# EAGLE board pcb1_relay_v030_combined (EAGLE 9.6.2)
2024-07-10 PCB made by JLCPCB.
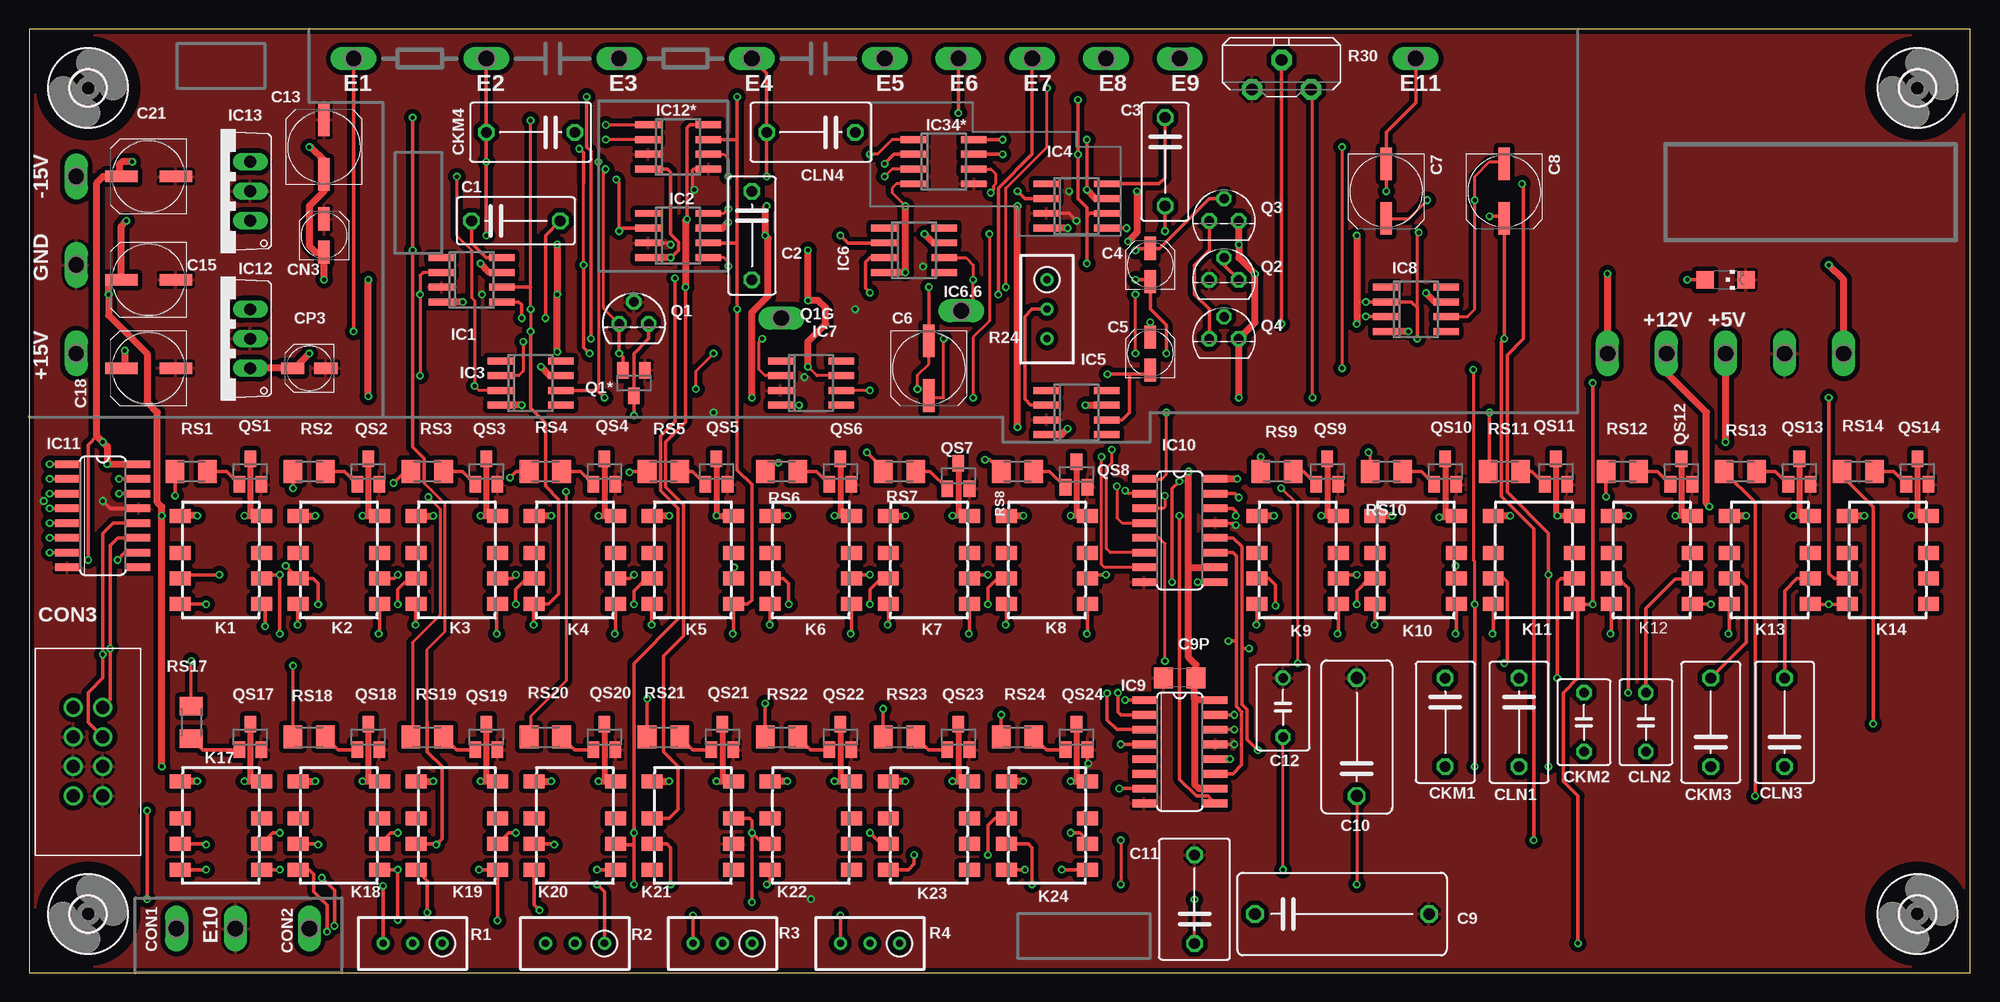
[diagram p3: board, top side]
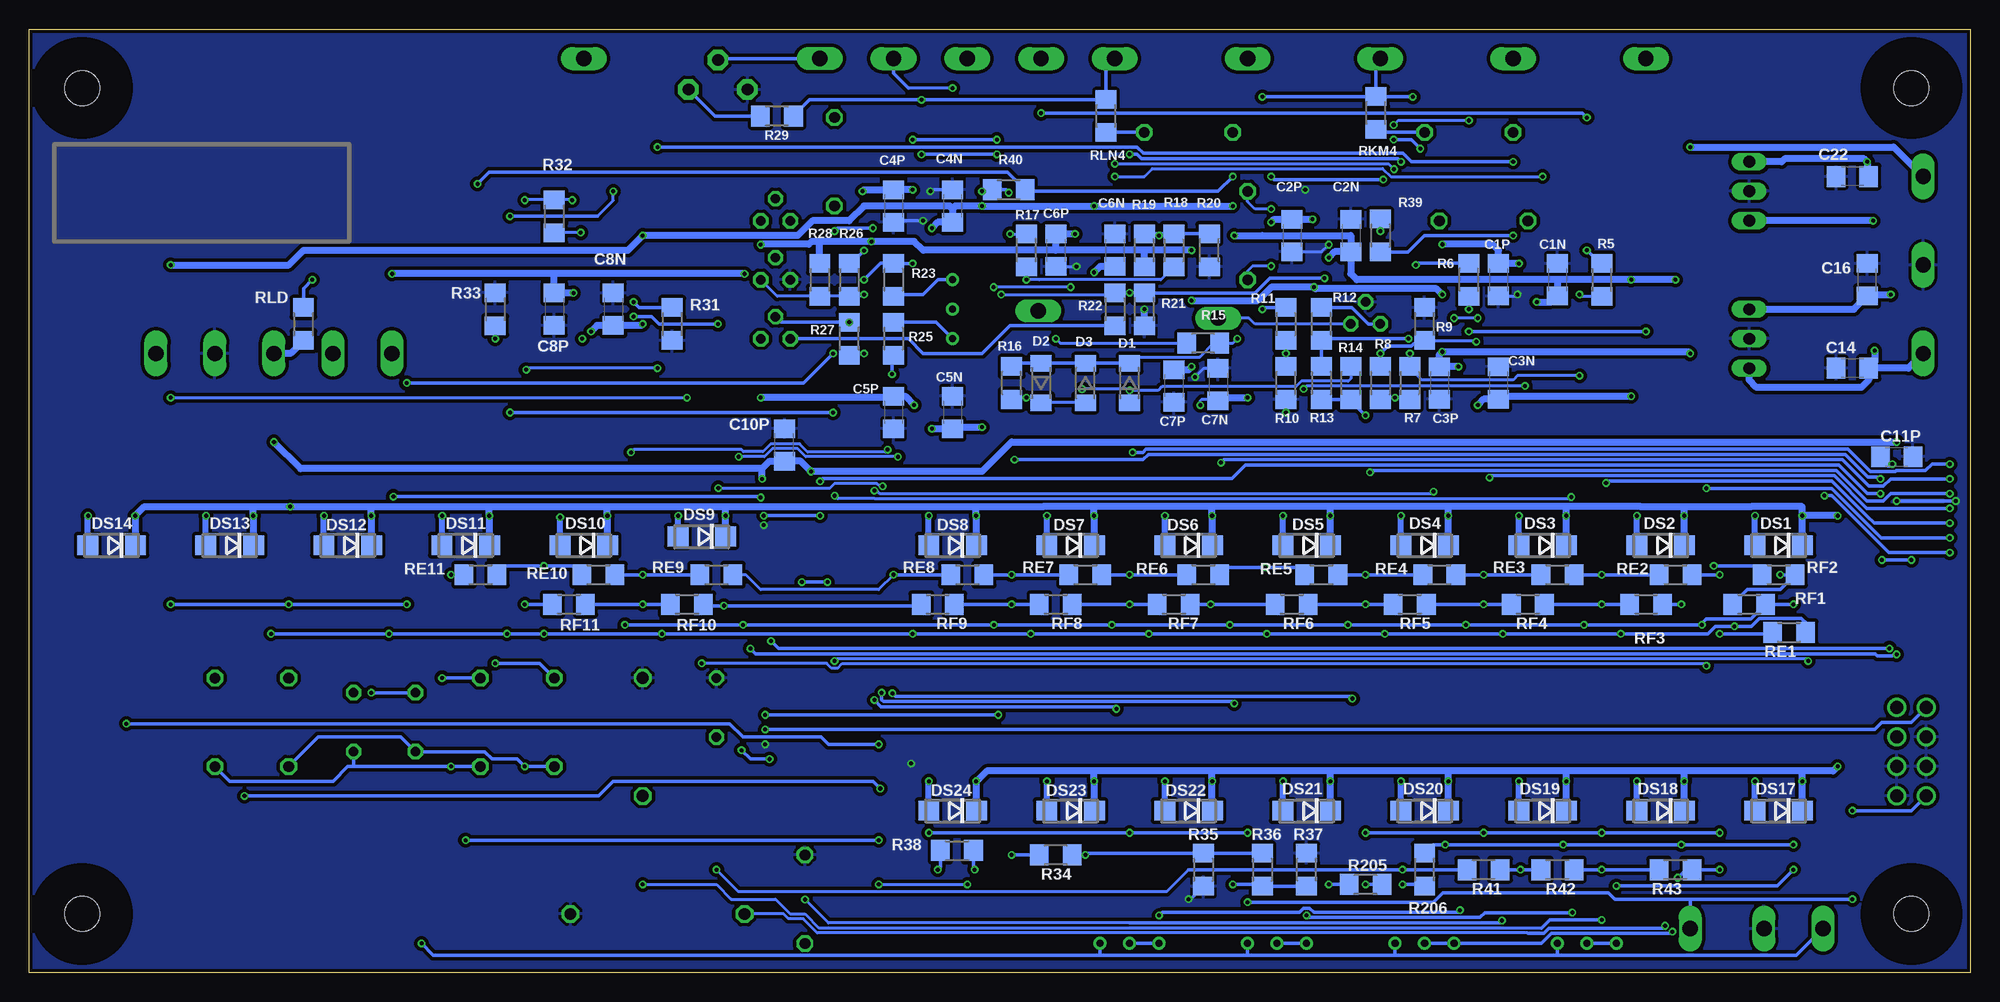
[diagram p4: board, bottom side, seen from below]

Size 167.13 x 81.28 mm. Coordinates in mm from the lower left corner, seen from the top.
Outline: 0,0 167.13,0 167.13,81.28 0,81.28 0,0
Copper layers (1*16): Top 0.035mm / dielectric 1.5mm / Bottom 0.035mm
Design rules "ITEADstudio_DRC for Eagle v6": minimum track width 6mil, minimum drill 12mil, track to track 6mil, track to pad 6mil, pad to pad 6mil, via to via 6mil, smd to smd 0mil, copper to edge 10mil, drill to drill 10mil, minimum pad ring 10mil, minimum via ring 6mil, stop-mask expansion 2mil, vias tented up to drill 100mil, thermal gap 10mil

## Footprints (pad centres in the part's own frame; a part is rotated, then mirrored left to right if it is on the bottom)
P1-13Y = drill 1.321 pad 1.905 long: TP 0,0
C075-042X103 = drill 0.914 octagon: 1 -3.81,0; 2 3.81,0
C1206 = smd 1.6 x 1.8: 1 -1.4,0; 2 1.4,0
UD-4X5,8_NICHICON = smd 2 x 1: + 1.425,0; - -1.425,0
UD-6,3X5,8_NICHICON = smd 2.8 x 1: + 2.35,0; - -2.35,0
C150-072X183 = drill 1.016 octagon: 1 -7.493,0; 2 7.493,0
C102-064X133 = drill 1.016 octagon: 1 -5.08,0; 2 5.08,0
C075-063X106 = drill 0.914 octagon: 1 -3.81,0; 2 3.81,0
C050-045X075 = drill 0.813 octagon: 1 -2.54,0; 2 2.54,0
C075-052X106 = drill 0.914 octagon: 1 -3.81,0; 2 3.81,0
61200821621 = drill 1.1: 1 -2.54,-1.27; 2 -2.54,1.27; 3 0,-1.27; 4 0,1.27; 5 2.54,-1.27; 6 2.54,1.27; 7 5.08,-1.27; 8 5.08,1.27
SOD80 = smd 1.4 x 1.8: 1 -1.7,0; 2 1.7,0
DO214AC = smd 1.8 x 1.7: A 2.05,0; C -2.05,0
SO08 = smd 0.6 x 2.2: 1 -1.905,-2.6; 2 -0.635,-2.6; 3 0.635,-2.6; 4 1.905,-2.6; 5 1.905,2.6; 6 0.635,2.6; 7 -0.635,2.6; 8 -1.905,2.6
SO16 = smd 0.66 x 2.032: 1 -4.445,-3.073; 2 -3.175,-3.073; 3 -1.905,-3.073; 4 -0.635,-3.073; 5 0.635,-3.073; 6 1.905,-3.073; 7 3.175,-3.073; 8 4.445,-3.073; 9 4.445,3.073; 10 3.175,3.073; 11 1.905,3.073; 12 0.635,3.073; 13 -0.635,3.073; 14 -1.905,3.073; 15 -3.175,3.073; 16 -4.445,3.073
TO220V = drill 1.016 long: 1 -2.54,-2.54; 2 0,-2.54; 3 2.54,-2.54
G6K-2F-Y = smd 1.2 x 1.8: 1 -3.8,-3.5; 2 -0.6,-3.5; 3 1.6,-3.5; 4 3.8,-3.5; 5 3.8,3.5; 6 1.6,3.5; 7 -0.6,3.5; 8 -3.8,3.5
CHIPLED_1206 = smd 1.5 x 1.5: A 0,-1.75; C 0,1.75
TO92G = drill 0.813 octagon: D -1.27,0; G 1.27,0; S 0,1.905
SOT23 = smd 1 x 1.4: 1 -0.95,-1.1; 2 0.95,-1.1; 3 0,1.1
TO92 = drill 0.813 octagon: 1 1.27,0; 2 0,1.905; 3 -1.27,0
RTRIM3296W = drill 0.61: 1 0,-2.54; 2 0,0; 3 0,2.54
R1206 = smd 1.6 x 1.803: 1 -1.422,0; 2 1.422,0
PT-10S = drill 1.016 pad 1.778 octagon: 1 -2.54,-1.27; 2 2.54,-1.27; 3 0,1.27
M1206 = smd 1.6 x 2: 1 -1.4,0; 2 1.4,0
3,0 = hole 3: 0,0

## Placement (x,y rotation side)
+5V  TPPAD1-13Y  [P1-13Y]  146.05,53.34 0 top
+12V  TPPAD1-13Y  [P1-13Y]  140.97,53.34 0 top
+15V  TPPAD1-13Y  [P1-13Y]  4.06,53.34 0 top
+15V1  TPPAD1-13Y  [P1-13Y]  135.89,53.34 0 top
-15V  TPPAD1-13Y  [P1-13Y]  4.06,68.58 0 top
-15V1  TPPAD1-13Y  [P1-13Y]  156.21,53.34 0 top
C1  15pF  [C075-042X103]  41.91,64.77 0 top
C1N  100n  [C1206]  35.56,59.69 270 bottom
C1P  100n  [C1206]  40.64,59.69 270 bottom
C2  22p  [C075-042X103]  62.23,63.5 270 top
C2N  100n  [C1206]  53.34,63.5 270 bottom
C2P  100n  [C1206]  58.42,63.5 270 bottom
C3  22p  [C075-042X103]  97.79,69.85 270 top
C3N  100n  [C1206]  40.64,50.8 270 bottom
C3P  100n  [C1206]  45.72,50.8 270 bottom
C4  10u/25V  [UD-4X5,8_NICHICON]  96.52,60.96 90 top
C4N  100n  [C1206]  87.63,66.04 270 bottom
C4P  100n  [C1206]  92.71,66.04 270 bottom
C5  10u/25V  [UD-4X5,8_NICHICON]  96.52,53.34 90 top
C5N  100n  [C1206]  87.63,48.26 270 bottom
C5P  100n  [C1206]  92.71,48.26 270 bottom
C6  100u/16V  [UD-6,3X5,8_NICHICON]  77.47,52.07 270 top
C6N  100n  [C1206]  73.66,62.23 270 bottom
C6P  100n  [C1206]  78.74,62.23 270 bottom
C7  100u/16V  [UD-6,3X5,8_NICHICON]  116.84,67.31 270 top
C7N  100n  [C1206]  64.77,50.67 270 bottom
C7P  100n  [C1206]  68.58,50.55 270 bottom
C8  100u/16V  [UD-6,3X5,8_NICHICON]  127,67.31 270 top
C8N  100n  [C1206]  116.84,57.15 270 bottom
C8P  100n  [C1206]  121.92,57.15 270 bottom
C9  1u  [C150-072X183]  113.03,5.08 0 top
C9P  100n  [C1206]  99.06,25.4 180 top
C10  470n  [C102-064X133]  114.3,20.32 90 top
C10P  100n  [C1206]  102.11,45.47 90 bottom
C11  100n  [C075-063X106]  100.33,6.35 90 top
C11P  100n  [C1206]  6.35,44.45 0 bottom
C12  10n  [C050-045X075]  107.95,22.86 90 top
C13  100u/16V  [UD-6,3X5,8_NICHICON]  25.4,71.12 90 top
C14  100n  [C1206]  10.16,52.07 180 bottom
C15  100u/16V  [UD-6,3X5,8_NICHICON]  10.29,59.69 180 top
C16  100n  [C1206]  8.89,59.69 90 bottom
C18  100u/16V  [UD-6,3X5,8_NICHICON]  10.29,52.07 180 top
C21  100u/16V  [UD-6,3X5,8_NICHICON]  10.29,68.58 180 top
C22  100n  [C1206]  10.16,68.58 180 bottom
CKM1  220n  [C075-052X106]  121.92,21.59 270 top
CKM2  22n  [C050-045X075]  133.86,21.59 270 top
CKM3  2n2  [C075-052X106]  144.78,21.59 90 top
CKM4  220p  [C075-052X106]  43.18,72.39 180 top
CLN1  220n  [C075-052X106]  128.27,21.59 270 top
CLN2  22n  [C050-045X075]  139.19,21.59 270 top
CLN3  2n2  [C075-052X106]  151.13,21.59 90 top
CLN4  220p  [C075-052X106]  67.31,72.39 180 top
CN3  1u/50V  [UD-4X5,8_NICHICON]  25.4,63.5 90 top
CON1  MAIN_OUT  [P1-13Y]  12.7,3.81 180 top
CON2  MAIN_OUT  [P1-13Y]  24.13,3.81 180 top
CON3  UC_IO  [61200821621]  5.08,17.78 90 top
CP3  1u/50V  [UD-4X5,8_NICHICON]  24.13,52.07 180 top
D1  1N4148  [SOD80]  72.39,50.8 270 bottom
D2  1N4148  [SOD80]  80.01,50.8 90 bottom
D3  1N4148  [SOD80]  76.2,50.8 270 bottom
DS1  M7  [DO214AC]  16.51,36.83 180 bottom
DS2  M7  [DO214AC]  26.67,36.83 180 bottom
DS3  M7  [DO214AC]  36.83,36.83 180 bottom
DS4  M7  [DO214AC]  46.99,36.83 180 bottom
DS5  M7  [DO214AC]  57.15,36.83 180 bottom
DS6  M7  [DO214AC]  67.31,36.83 180 bottom
DS7  M7  [DO214AC]  77.47,36.83 180 bottom
DS8  M7  [DO214AC]  87.63,36.83 180 bottom
DS9  M7  [DO214AC]  109.22,37.59 180 bottom
DS10  M7  [DO214AC]  119.38,36.83 180 bottom
DS11  M7  [DO214AC]  129.54,36.83 180 bottom
DS12  M7  [DO214AC]  139.7,36.83 180 bottom
DS13  M7  [DO214AC]  149.86,36.83 180 bottom
DS14  M7  [DO214AC]  160.02,36.83 180 bottom
DS17  M7  [DO214AC]  16.51,13.97 180 bottom
DS18  M7  [DO214AC]  26.67,13.97 180 bottom
DS19  M7  [DO214AC]  36.83,13.97 180 bottom
DS20  M7  [DO214AC]  46.99,13.97 180 bottom
DS21  M7  [DO214AC]  57.15,13.97 180 bottom
DS22  M7  [DO214AC]  67.31,13.97 180 bottom
DS23  M7  [DO214AC]  77.47,13.97 180 bottom
DS24  M7  [DO214AC]  87.63,13.97 180 bottom
E1  TPPAD1-13Y  [P1-13Y]  27.94,78.74 90 top
E2  TPPAD1-13Y  [P1-13Y]  39.37,78.74 90 top
E3  TPPAD1-13Y  [P1-13Y]  50.8,78.74 90 top
E4  TPPAD1-13Y  [P1-13Y]  62.23,78.74 90 top
E5  TPPAD1-13Y  [P1-13Y]  73.66,78.74 90 top
E6  TPPAD1-13Y  [P1-13Y]  80.01,78.74 90 top
E7  TPPAD1-13Y  [P1-13Y]  86.36,78.74 90 top
E8  TPPAD1-13Y  [P1-13Y]  92.71,78.74 90 top
E9  TPPAD1-13Y  [P1-13Y]  99.06,78.74 270 top
E10  MAIN_OUT  [P1-13Y]  17.78,3.81 0 top
E11  TPPAD1-13Y  [P1-13Y]  119.38,78.74 90 top
GND  TPPAD1-13Y  [P1-13Y]  4.06,60.96 0 top
GND1  TPPAD1-13Y  [P1-13Y]  151.13,53.34 0 top
IC1  NE5534D  [SO08]  38.1,59.69 270 top
IC2  NE5534D  [SO08]  55.88,63.5 270 top
IC3  NE5534D  [SO08]  43.18,50.8 270 top
IC4  NE5534D  [SO08]  90.17,66.04 270 top
IC5  LM318D  [SO08]  90.17,48.26 270 top
IC6  LM318D  [SO08]  76.2,62.23 270 top
IC6.6  TPPAD1-13Y  [P1-13Y]  80.26,57.02 90 top
IC7  LM318D  [SO08]  67.31,50.8 270 top
IC8  NE5534D  [SO08]  119.38,57.15 270 top
IC9  74HC595D  [SO16]  99.06,19.05 270 top
IC10  74HC595D  [SO16]  99.06,38.1 270 top
IC11  74HC595D  [SO16]  6.35,39.37 270 top
IC12  7812TV  [TO220V]  16.51,54.61 90 top
IC12*  OPA1612  [SO08]  55.88,71.12 270 top
IC13  7805TV  [TO220V]  16.51,67.31 90 top
IC34*  OPA1612D  [SO08]  78.74,69.85 270 top
K1  G6K-2F-Y  [G6K-2F-Y]  16.51,35.56 270 top
K2  G6K-2F-Y  [G6K-2F-Y]  26.67,35.56 270 top
K3  G6K-2F-Y  [G6K-2F-Y]  36.83,35.56 270 top
K4  G6K-2F-Y  [G6K-2F-Y]  46.99,35.56 270 top
K5  G6K-2F-Y  [G6K-2F-Y]  57.15,35.56 270 top
K6  G6K-2F-Y  [G6K-2F-Y]  67.31,35.56 270 top
K7  G6K-2F-Y  [G6K-2F-Y]  77.47,35.56 270 top
K8  G6K-2F-Y  [G6K-2F-Y]  87.63,35.56 270 top
K9  G6K-2F-Y  [G6K-2F-Y]  109.22,35.56 270 top
K10  G6K-2F-Y  [G6K-2F-Y]  119.38,35.56 270 top
K11  G6K-2F-Y  [G6K-2F-Y]  129.54,35.56 270 top
K12  G6K-2F-Y  [G6K-2F-Y]  139.7,35.56 270 top
K13  G6K-2F-Y  [G6K-2F-Y]  149.86,35.56 270 top
K14  G6K-2F-Y  [G6K-2F-Y]  160.02,35.56 270 top
K17  G6K-2F-Y  [G6K-2F-Y]  16.51,12.7 270 top
K18  G6K-2F-Y  [G6K-2F-Y]  26.67,12.7 270 top
K19  G6K-2F-Y  [G6K-2F-Y]  36.83,12.7 270 top
K20  G6K-2F-Y  [G6K-2F-Y]  46.99,12.7 270 top
K21  G6K-2F-Y  [G6K-2F-Y]  57.15,12.7 270 top
K22  G6K-2F-Y  [G6K-2F-Y]  67.31,12.7 270 top
K23  G6K-2F-Y  [G6K-2F-Y]  77.47,12.7 270 top
K24  G6K-2F-Y  [G6K-2F-Y]  87.63,12.7 270 top
LED1  LD1  [CHIPLED_1206]  146.05,59.69 270 top
Q1  PN4091  [TO92G]  52.07,55.88 0 top
Q1*  MMBF4091  [SOT23]  52.07,50.8 180 top
Q1G  TPPAD1-13Y  [P1-13Y]  64.77,56.39 90 top
Q2  2N3904  [TO92]  102.87,59.69 0 top
Q3  2N3904  [TO92]  102.87,64.77 0 top
Q4  2N3904  [TO92]  102.87,54.61 0 top
QS1  SS8050  [SOT23]  19.05,43.18 0 top
QS2  SS8050  [SOT23]  29.21,43.18 0 top
QS3  SS8050  [SOT23]  39.37,43.18 0 top
QS4  SS8050  [SOT23]  49.53,43.18 0 top
QS5  SS8050  [SOT23]  59.18,43.18 0 top
QS6  SS8050  [SOT23]  69.85,43.18 0 top
QS7  SS8050  [SOT23]  80.01,42.8 0 top
QS8  SS8050  [SOT23]  90.17,42.93 0 top
QS9  SS8050  [SOT23]  111.76,43.18 0 top
QS10  SS8050  [SOT23]  121.92,43.18 0 top
QS11  SS8050  [SOT23]  131.44,43.18 0 top
QS12  SS8050  [SOT23]  142.24,43.18 0 top
QS13  SS8050  [SOT23]  152.4,43.18 0 top
QS14  SS8050  [SOT23]  162.56,43.18 0 top
QS17  SS8050  [SOT23]  19.05,20.32 0 top
QS18  SS8050  [SOT23]  29.21,20.32 0 top
QS19  SS8050  [SOT23]  39.37,20.32 0 top
QS20  SS8050  [SOT23]  49.53,20.32 0 top
QS21  SS8050  [SOT23]  59.69,20.32 0 top
QS22  SS8050  [SOT23]  69.85,20.32 0 top
QS23  SS8050  [SOT23]  80.01,20.32 0 top
QS24  SS8050  [SOT23]  90.17,20.32 0 top
R1  5K  [RTRIM3296W]  33.02,2.54 90 top
R2  5K  [RTRIM3296W]  46.99,2.54 90 top
R3  5K  [RTRIM3296W]  59.69,2.54 90 top
R4  5K  [RTRIM3296W]  72.39,2.54 90 top
R5  6K8  [R1206]  31.75,59.69 90 bottom
R6  10k  [R1206]  43.18,59.69 270 bottom
R7  150k  [R1206]  48.26,50.8 90 bottom
R8  560  [R1206]  50.8,50.8 90 bottom
R9  330  [R1206]  46.99,55.88 270 bottom
R10  270  [R1206]  58.93,50.8 270 bottom
R11  10k  [R1206]  58.93,55.88 90 bottom
R12  1K5  [R1206]  55.88,55.88 270 bottom
R13  750k  [R1206]  55.88,50.8 90 bottom
R14  10k  [R1206]  53.34,50.8 270 bottom
R15  10k  [R1206]  66.04,54.23 0 bottom
R16  100k  [R1206]  82.55,50.8 270 bottom
R17  1k  [R1206]  81.28,62.23 270 bottom
R18  10k  [R1206]  68.58,62.23 90 bottom
R19  6K8  [R1206]  71.12,62.23 270 bottom
R20  1K3  [R1206]  65.53,62.23 270 bottom
R21  1M  [R1206]  71.12,57.15 270 bottom
R22  10k  [R1206]  73.66,57.15 90 bottom
R23  10k  [R1206]  92.71,59.69 90 bottom
R24  1K  [RTRIM3296W]  87.63,57.15 180 top
R25  10k  [R1206]  92.71,54.61 90 bottom
R26  10k  [R1206]  96.52,59.69 90 bottom
R27  10k  [R1206]  96.52,54.61 270 bottom
R28  22K  [R1206]  99.06,59.69 90 bottom
R29  5K6  [R1206]  102.74,73.79 0 bottom
R30  2K5  [PT-10S]  107.82,77.34 0 top
R31  1k  [R1206]  111.76,55.88 90 bottom
R32  2K2  [R1206]  121.92,65.15 90 bottom
R33  100k  [R1206]  127,57.15 90 bottom
R34  2K  [R1206]  78.74,10.16 0 bottom
R35  1K3  [R1206]  66.04,8.89 90 bottom
R36  1K8  [R1206]  60.96,8.89 90 bottom
R37  820  [R1206]  57.15,8.89 270 bottom
R38  620  [R1206]  87.25,10.54 180 bottom
R39  220  [R1206]  50.8,63.5 90 bottom
R40  220  [R1206]  82.8,67.44 180 bottom
R41  1M  [R1206]  41.91,8.89 0 bottom
R42  1M  [R1206]  35.56,8.89 0 bottom
R43  1M  [R1206]  25.4,8.89 0 bottom
R205  2M7  [R1206]  52.07,7.62 0 bottom
R206  22K  [R1206]  46.99,8.89 270 bottom
RE1  7K5  [R1206]  15.62,29.34 180 bottom
RE2  5K62  [R1206]  25.4,34.29 180 bottom
RE3  6K19  [R1206]  35.56,34.29 180 bottom
RE4  3K83  [R1206]  45.72,34.29 180 bottom
RE5  3K48  [R1206]  55.88,34.29 180 bottom
RE6  2K15  [R1206]  66.04,34.29 180 bottom
RE7  1K96  [R1206]  76.2,34.29 180 bottom
RE8  1K78  [R1206]  86.36,34.29 180 bottom
RE9  1K1  [R1206]  107.95,34.29 180 bottom
RE10  1K  [R1206]  118.11,34.29 180 bottom
RE11  3K83  [R1206]  128.27,34.29 180 bottom
RF1  7K5  [R1206]  19.05,31.75 180 bottom
RF2  5K62  [R1206]  16.51,34.29 180 bottom
RF3  6K19  [R1206]  27.94,31.75 180 bottom
RF4  3K83  [R1206]  38.1,31.75 180 bottom
RF5  3K48  [R1206]  48.26,31.75 180 bottom
RF6  2K15  [R1206]  58.42,31.75 180 bottom
RF7  1K96  [R1206]  68.58,31.75 180 bottom
RF8  1K78  [R1206]  78.74,31.75 180 bottom
RF9  1K1  [R1206]  88.9,31.75 180 bottom
RF10  1K  [R1206]  110.49,31.75 180 bottom
RF11  3K83  [R1206]  120.65,31.75 180 bottom
RKM4  330  [R1206]  51.18,74.04 270 bottom
RLD  3K9  [R1206]  143.51,55.88 90 bottom
RLN4  330  [R1206]  74.42,73.79 270 bottom
RS1  4k7  [M1206]  13.97,43.18 180 top
RS2  4k7  [M1206]  24.13,43.18 180 top
RS3  4k7  [M1206]  34.29,43.18 180 top
RS4  4k7  [M1206]  44.45,43.18 180 top
RS5  4k7  [M1206]  54.61,43.18 180 top
RS6  4k7  [M1206]  64.77,43.18 180 top
RS7  4k7  [M1206]  74.93,43.18 180 top
RS8  4k7  [M1206]  85.09,43.18 180 top
RS9  4k7  [M1206]  107.44,43.18 180 top
RS10  4k7  [M1206]  116.84,43.18 180 top
RS11  4k7  [M1206]  127,43.18 180 top
RS12  4k7  [M1206]  137.16,43.18 180 top
RS13  4k7  [M1206]  147.32,43.18 180 top
RS14  4k7  [M1206]  157.48,43.18 180 top
RS17  4k7  [M1206]  13.97,21.59 90 top
RS18  4k7  [M1206]  24.13,20.32 180 top
RS19  4k7  [M1206]  34.29,20.32 180 top
RS20  4k7  [M1206]  44.45,20.32 180 top
RS21  4k7  [M1206]  54.61,20.32 180 top
RS22  4k7  [M1206]  64.77,20.32 180 top
RS23  4k7  [M1206]  74.93,20.32 180 top
RS24  4k7  [M1206]  85.09,20.32 180 top
U$1  [3,0]  5.08,5.08 0 top
U$2  [3,0]  5.08,76.2 0 top
U$3  [3,0]  162.56,76.2 0 top
U$4  [3,0]  162.56,5.08 0 top

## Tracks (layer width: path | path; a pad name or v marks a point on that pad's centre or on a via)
+5V  (via drill 0.35)
  Top 0.305: IC11.10 8.26,36.2 v7.62,35.56 | v5.08,35.56 5.08,45.47 5.84,46.23
  Top 0.61: v8.89,69.85 8,69.85 7.75,69.6 7.75,68.77 C21.+ 6.35,68.58 5.84,68.07 5.84,46.23 v6.35,45.72 6.73,45.34 v6.73,43.81 IC11.16 | IC9.16 100.33,23.5 | 99.82,34.92 IC10.10 | 99.82,34.92 99.82,27.18 100.46,26.54 C9P.1 100.33,25.27 100.33,23.5 | 99.82,34.92 v99.82,43.18 | v104.01,42.55 IC10.16 | IC9.10 100.71,15.88 100.33,16.26 100.33,23.5 | v146.05,45.72 +5V.TP
  Bottom 0.305: v7.62,35.56 v5.08,35.56
  Bottom 0.61: C22.1 8.89,68.71 v8.89,69.85 9.14,70.1 16,70.1 16.26,69.85 IC13.3 | C11P.1 7.12,43.81 v6.73,43.81 | v6.35,45.72 82.55,45.72 85.09,43.18 v99.82,43.18 100.71,44.07 C10P.1 103.38,44.07 104.01,43.43 | v104.01,42.55 104.01,43.43 | 104.01,43.43 143.76,43.43 v146.05,45.72 | RLD.1 144.63,53.34 +5V.TP
+12V  (via drill 0.35)
  Top 0.61: v8.38,64.77 7.94,64.33 C15.+ 7.24,59.69 6.86,59.31 v6.86,58.42 6.86,56.64 10.16,53.34 10.16,49.15 11.05,48.26 11.05,40.51 11.43,40.13 v11.43,39.37 v11.43,17.78 | v14.48,39.37 K1.1 | K6.1 63.93,39.24 64.05,39.37 v65.28,39.37 | K8.1 v85.6,39.37 | v107.19,39.37 107.18,39.36 K9.1 | v117.35,39.37 117.34,39.36 K10.1 | v127.51,39.37 127.5,39.36 K11.1 | v137.67,39.37 137.66,39.36 K12.1 | v147.83,39.37 147.82,39.36 K13.1 | v157.99,39.37 157.98,39.36 K14.1 | v14.48,16.51 K17.1 | v65.28,16.51 K22.1 | v75.44,16.51 75.43,16.5 K23.1 | v85.6,16.51 85.59,16.5 K24.1 | K4.1 v44.96,39.37 | v55.12,39.37 55.11,39.36 K5.1 | K21.1 v55.12,16.51 | K7.1 75.43,39.36 v75.44,39.37 | K20.1 44.95,16.5 v44.96,16.51 | K3.1 34.79,39.36 v34.8,39.37 | K19.1 34.79,16.5 v34.8,16.51 | K18.1 24.63,16.5 v24.64,16.51 | K2.1 24.63,39.36 v24.64,39.37 | v144.65,40.16 144.4,40.41 144.4,48.26 140.97,51.69 +12V.TP
  Bottom 0.61: IC12.3 10.03,57.15 C16.1 8.76,58.42 v6.86,58.42 | v8.38,64.77 IC13.1 | DS1.C 14.46,39.35 | 14.46,39.35 v14.48,39.37 14.48,40.16 18.87,40.16 18.89,40.13 24.64,40.13 | DS9.C 107.17,39.35 v107.19,39.37 107.19,40.03 107.31,40.16 | DS10.C 117.33,39.35 v117.35,39.37 117.35,40.16 | DS11.C 127.49,39.35 v127.51,39.37 127.51,40.16 | DS12.C 137.65,39.35 v137.67,39.37 137.67,40.16 | DS13.C 147.81,39.35 v147.83,39.37 147.83,40.03 147.96,40.16 | DS14.C 157.97,39.35 v157.99,39.37 157.2,40.16 147.96,40.16 | DS17.C 14.46,16.49 v14.48,16.51 14.48,17.4 | DS22.C 65.28,13.99 v65.28,16.51 65.28,17.4 | DS23.C 75.42,16.49 v75.44,16.51 75.44,17.27 75.56,17.4 | DS24.C 85.58,16.49 | 85.58,16.49 v85.6,16.51 | DS5.C 55.1,39.35 v55.12,39.37 55.12,40.03 55.24,40.16 | 85.58,16.49 84.67,17.4 75.56,17.4 | 14.48,17.4 11.81,17.4 v11.43,17.78 | 14.48,17.4 24.64,17.4 | 24.64,17.4 34.8,17.4 | 34.8,17.4 44.96,17.4 | 44.96,17.4 55.12,17.4 | 55.12,17.4 65.28,17.4 | 65.28,17.4 75.56,17.4 | 34.8,40.16 28.38,40.16 28.35,40.13 24.64,40.13 | 34.8,40.16 44.96,40.16 | 44.96,40.16 55.24,40.16 | 55.24,40.16 65.28,40.16 | 65.28,40.16 75.44,40.16 | 75.44,40.16 79.83,40.16 79.85,40.13 85.6,40.13 | 147.96,40.16 v144.65,40.16 137.67,40.16 | 137.67,40.16 127.51,40.16 | 127.51,40.16 117.35,40.16 | 117.35,40.16 107.31,40.16 | 107.31,40.16 85.62,40.16 85.6,40.13 | v11.43,39.37 14.44,39.37 14.46,39.35 | DS21.C 55.1,16.49 v55.12,16.51 55.12,17.4 | 65.28,40.16 v65.28,39.37 65.26,39.35 DS6.C | DS7.C 75.42,39.35 v75.44,39.37 75.44,40.16 | DS8.C 85.58,39.35 v85.6,39.37 85.6,40.13 | DS20.C 44.94,16.49 v44.96,16.51 44.96,17.4 | DS3.C 34.8,36.85 v34.8,39.37 34.8,40.16
  Bottom 0.61: DS19.C 34.78,16.49 v34.8,16.51 34.8,17.4 | DS18.C 24.62,16.49 v24.64,16.51 24.64,17.4 | DS2.C 24.62,39.35 v24.64,39.37 24.64,40.13 | DS4.C 44.94,39.35 v44.96,39.37 44.96,40.16
+15V  (via drill 0.35)
  Top 0.254: IC7.7 67.82,51.44 v67.06,52.2
  Top 0.305: K21.2 55.08,13.3 55.88,14.1 55.88,17.78 54.61,19.05 54.61,27.29 56.34,29.02 56.34,40.31 54.81,41.83 54.81,45.72 56.52,47.42 v56.52,59.05 | IC34*.8 v83.82,71.75 | v91.06,71.75 v91.06,67.44 | IC12*.8 56.9,73.03 56.64,72.77 v56.64,64.9
  Top 0.61: IC2.7 59.69,64.14 v60.2,64.64 | IC1.7 39.62,60.33 v38.86,61.09 | IC3.7 44.83,51.44 v44.07,52.2 | IC6.7 77.85,62.87 v77.09,63.63 | IC4.7 91.82,66.67 v91.06,67.44 | v90.93,48.9 IC5.7 | IC8.7 121.03,57.78 v120.27,58.55 | IC12.1 CP3.+ 22.86,52.07 v24.13,53.34 | v95.38,67.31 95.38,63.75 v94.61,62.99 | Q3.1 v104.14,62.72 104.14,61.59 v105.54,60.2 105.54,56.01 Q4.1 v104.14,49.53 | v67.06,62.23 v67.06,57.91 67.94,57.91 68.58,57.28 68.58,55.88 67.06,54.36 v67.06,52.2 | v56.64,64.9 56.52,64.77 v56.52,59.05 | v45.47,53.48 v45.47,58.42 v45.47,62.74 | v8.26,53.59 8.26,52.39 C18.+ | v135.89,60.2 +15V1.TP
  Bottom 0.305: v83.82,71.75 v91.06,71.75
  Bottom 0.61: v60.2,64.64 59.94,64.9 C2P.1 v56.65,64.9 v56.64,64.9 | v38.86,61.09 C1P.1 40.64,62.23 41.15,62.74 v45.47,62.74 | v44.07,52.2 C3P.1 45.72,53.23 v45.47,53.48 24.27,53.48 v24.13,53.34 | v77.09,63.63 C6P.1 | C6P.1 | v91.06,67.44 C4P.1 | C4P.1 | v90.93,48.9 91.7,49.66 C5P.1 92.84,49.53 v104.14,49.53 | v120.27,58.55 C8P.1 121.92,60.2 | C14.1 8.76,51.06 9.4,50.42 18.41,50.42 19.05,51.05 IC12.1 | R19.2 71.12,62.23 | 71.12,62.23 78.74,62.23 | 78.74,62.23 90.17,62.23 90.93,62.99 v94.61,62.99 99.06,62.99 | v95.38,67.31 95.25,67.44 C4P.1 | 99.06,62.99 99.76,62.99 100.01,62.74 104.14,62.74 v104.14,62.72 | v105.54,60.2 121.92,60.2 | R28.2 99.06,62.99 | v67.06,62.23 71.12,62.23 | v45.47,58.42 45.97,58.93 56.39,58.93 v56.52,59.05 60.2,59.05 61.34,57.91 v67.06,57.91 | v8.26,53.59 8.26,52.58 C14.1 | +15V.TP 5.33,52.07 C14.1 | 78.74,62.23 C6P.1 | 121.92,60.2 v135.89,60.2 | C7P.1 67.31,51.95 v67.06,52.2
-15V  (via drill 0.35)
  Top 0.254: IC7.4 v66.29,48.9 | IC34*.4 74.68,67.94 74.3,67.56 74.3,67.18 v75.44,66.04
  Top 0.305: IC12*.4 54.99,69.22 55.24,68.96 55.24,63.61 55.91,62.95 55.91,62.23 55.27,61.59 v55.24,61.59
  Top 0.61: v55.24,61.59 IC2.4 | v37.34,57.78 IC1.4 | v42.42,48.9 IC3.4 | IC6.4 v75.44,60.33 v75.44,66.04 | v89.41,64.14 IC4.4 | IC5.4 88.9,46.35 v89.41,46.86 | v118.75,55.24 IC8.4 | v25.4,59.69 CN3.- 24.67,62.08 24.13,62.61 24.13,66.04 25.4,67.31 C13.- 25.4,69.98 24.26,71.12 v24.13,71.12 | v29.21,49.66 v29.21,59.69 | v85.09,46.99 v85.09,66.04 | v114.3,63.5 v114.3,55.88 | v63.5,66.04 63.37,65.91 v63.37,63.5 63.63,63.25 63.63,58.29 62.23,56.9 v62.23,49.53 | -15V1.TP 156.21,59.69 v154.94,60.96
  Bottom 0.254: v66.29,48.9 66.29,49.28 66.17,49.4 64.9,49.4 C7N.2
  Bottom 0.61: C2N.2 54.74,62.1 v55.24,61.59 | v42.42,48.9 41.91,49.4 C3N.2 40.38,49.66 v29.21,49.66 | C6N.2 74.93,60.83 v75.44,60.33 | v89.41,64.14 88.9,64.64 C4N.2 87.63,65.79 | v89.41,46.86 C5N.2 87.5,46.99 v85.09,46.99 | v118.75,55.24 118.24,55.75 C8N.2 114.43,55.75 v114.3,55.88 | 87.63,65.79 87.38,66.04 v85.09,66.04 v75.44,66.04 v63.5,66.04 | v63.37,63.5 60.96,63.5 53.34,63.5 C2N.2 | C2N.2 53.34,60.2 52.83,59.69 35.56,59.69 | 35.56,59.69 C1N.2 36.06,57.78 v37.34,57.78 | v24.13,71.12 6.6,71.12 -15V.TP | C7N.2 64.51,49.53 v62.23,49.53 | v25.4,59.69 v29.21,59.69 35.56,59.69 | 87.63,65.79 87.88,66.04 95.25,66.04 96.52,64.77 99.69,64.77 100.97,63.5 v114.3,63.5 115.57,62.23 143.51,62.23 144.78,60.96 v154.94,60.96
E1  (via drill 0.35)
  Top 0.254: v43.18,55.24 v43.18,57.15 43.18,59.05 v43.18,73.41 | v49.66,73.02 v49.66,73.03 IC12*.1
  Top 0.305: v15.24,31.75 v15.23,31.76 K1.4 | v23.11,29.97 23.11,31.7 K2.4 | v33.27,29.97 33.27,31.7 K3.4 | v43.43,29.97 43.43,31.7 K4.4 44.71,31.76 45.59,32.64 45.59,40.77 44.45,41.91 44.45,47.37 43.18,48.64 v43.18,55.24 | K5.4 53.59,31.7 v53.59,29.97 | v63.75,29.97 63.81,30.03 K6.4 | v73.91,29.97 73.97,30.03 K7.4 | v84.07,29.97 84.13,30.03 K8.4 | v105.66,29.97 105.72,30.03 K9.4 | v115.82,29.97 115.88,30.03 K10.4 | v27.94,55.24 E1.TP | IC1.6 43.18,59.05
  Bottom 0.254: v43.18,57.15 R6.2 | v43.18,73.41 49.27,73.41 v49.66,73.02
  Bottom 0.305: v23.11,29.97 23.24,29.97 | 23.24,29.97 v33.27,29.97 v43.43,29.97 v53.59,29.97 v63.75,29.97 v73.91,29.97 v84.07,29.97 v105.66,29.97 v115.82,29.97 | v15.24,31.75 RF1.1 18.9,30.48 22.73,30.48 23.24,29.97 | v43.18,55.24 v27.94,55.24
E2  (via drill 0.35)
  Top 0.254: v124.46,31.75 124.46,35.43 124.33,35.56 v124.33,51.94 | v113.03,71.12 v113.03,52.07
  Top 0.305: v124.46,31.75 v124.46,17.78 | E2.TP CKM4.2 v39.37,69.85 v39.37,63.5
  Bottom 0.254: v113.03,52.07 124.21,52.07 v124.33,51.94
  Bottom 0.305: RF11.2 v124.46,31.75 | R39.1 48.41,62.08 46.99,63.5 v39.37,63.5 | CKM3.1 142.24,20.32 135.13,20.32 CKM2.2 127.89,19.05 127.26,18.42 125.1,18.42 v124.46,17.78 CKM1.2 | v113.03,71.12 71.74,71.12 71.19,70.57 48.85,70.57 48.39,70.11 48.13,69.85 v39.37,69.85
E3  (via drill 0.35)
  Top 0.305: K1.5 20.32,31.45 v20.32,29.84 | v30.1,29.21 30.17,29.28 K2.5 | v40.26,29.21 40.26,31.69 K3.5 | v50.42,29.21 50.49,29.28 K4.5 | v60.58,29.21 60.65,29.28 K5.5 61.86,31.76 62.23,32.13 62.23,42.04 60.96,43.31 v60.96,57.15 60.96,60.1 60.96,62.87 | v70.74,29.21 70.81,29.28 K6.5 | v80.9,29.21 80.97,29.28 K7.5 | v91.06,29.21 91.13,29.28 K8.5 | v112.65,29.21 112.72,29.28 K9.5 | v122.81,29.21 122.88,29.28 K10.5 | v125.98,29.21 126.04,29.27 K11.4 | v136.14,29.21 136.2,29.27 K12.4 | v146.3,29.21 146.36,29.27 K13.4 | v60.96,75.44 60.96,72.39 60.96,71.75 | v48.01,75.44 48.01,71.11 48.37,70.75 v48.37,54.61 | 60.96,71.75 60.96,62.87 | IC2.6 60.96,62.87 | IC12*.7 60.96,71.75
  Bottom 0.305: v146.3,29.21 v136.14,29.21 v125.98,29.21 v122.81,29.21 v112.65,29.21 v91.06,29.21 v80.9,29.21 v70.74,29.21 v60.58,29.21 v50.42,29.21 v40.26,29.21 v30.1,29.21 22.61,29.21 21.97,29.84 v20.32,29.84 18.89,29.84 18.19,30.54 14.54,30.54 14.1,30.1 14.2,30 RE1.1 | v60.96,57.15 60.81,57.3 R11.2 | R13.2 R12.2 55.73,54.61 v48.37,54.61 | RKM4.1 51.18,78.36 E3.TP | v60.96,75.44 60.94,75.46 RKM4.1 | v48.01,75.44 48.03,75.46 RKM4.1
E4  (via drill 0.35)
  Top 0.305: v128.52,67.94 128.65,67.82 128.65,54.61 127.25,53.21 127.25,41.4 130.81,37.85 v130.81,34.29 v130.81,17.78 | v63.5,68.58 CLN4.2 63.5,77.47 E4.TP
  Bottom 0.305: CLN2.2 139.19,17.78 | v130.81,34.29 RE11.2 | v128.52,67.94 127.51,68.96 82.91,68.96 R40.1 81.25,67.31 64.77,67.31 v63.5,68.58 | CLN1.2 v130.81,17.78 139.19,17.78 | 139.19,17.78 139.7,17.78 140.97,16.51 149.86,16.51 CLN3.1
E5  (via drill 0.35)
  Top 0.305: K13.5 v154.94,31.75 K14.4 | v144.78,31.75 v144.77,31.76 K12.5 | 133.35,31.75 v134.62,31.75 v134.62,50.8 | 133.35,31.75 K11.5 | v97.9,53.34 97.9,55.77 96.52,57.15 C4.- 96.36,59.69 v95.25,59.69 | IC4.6 91.31,65.41 91.06,65.15 | 91.06,65.15 v91.06,61.09 | 91.06,65.15 91.06,65.91 90.3,66.67 v90.3,70.48 v90.3,75.18 | v48.9,7.62 49.53,6.99 R2.1 | v133.35,2.54 133.35,15.24 132.08,16.51 132.08,24.13 133.35,25.4 133.35,31.75 | IC34*.7 v83.82,70.49
  Bottom 0.305: v154.94,31.75 v144.78,31.75 v134.62,31.75 | v134.62,50.8 100.44,50.8 v97.9,53.34 | v95.25,59.69 93.83,61.11 R23.2 92.69,61.09 v91.06,61.09 | CON1.TP 14.99,1.52 35.56,1.52 | v48.9,7.62 47.14,7.62 R206.2 | v133.35,2.54 132.33,1.52 74.93,1.52 | 35.56,1.52 49.53,1.52 | 49.53,1.52 62.23,1.52 | 62.23,1.52 74.93,1.52 | R1.1 35.56,1.52 | R2.1 49.53,1.52 | R3.1 62.23,1.52 | R4.1 74.93,1.52 | E5.TP 74.42,77.98 RLN4.1 74.45,75.18 v90.3,75.18 99.92,75.18 R29.2 | v83.82,70.49 v90.29,70.49 v90.3,70.48
E6  (via drill 0.35)
  Top 0.254: 33.99,42.2 34.61,41.59 34.62,41.59 35.81,40.4 35.81,29.4 34.29,27.87 34.29,21.59
  Top 0.305: K17.3 15.19,11.1 v15.24,11.05 | v24.89,11.05 24.84,11.1 K18.3 | K19.3 35,11.1 v35.05,11.05 35.56,11.56 35.56,17.78 34.29,19.05 34.29,21.59 | v45.21,11.05 45.16,11.1 K20.3 | 33.99,42.2 33.99,44.31 33.02,45.28 v33.02,62.23 v33.02,73.66 | v80.01,74.04 E6.TP
  Bottom 0.305: v15.24,11.05 v24.89,11.05 v35.05,11.05 v45.21,11.05 46.25,11.05 R206.1 | v33.02,62.23 31.9,61.11 R5.2 | v33.02,73.66 33.4,74.04 v80.01,74.04
E7  (via drill 0.35)
  Top 0.305: K17.6 20.98,12.06 v21.59,12.06 | v31.75,12.06 31.14,12.06 K18.6 | v41.91,12.06 41.3,12.06 K19.6 | v52.07,7.62 52.07,11.05 | 52.07,11.05 v52.07,12.06 52.07,26.67 55.88,30.48 55.88,40.01 54.36,41.53 54.36,46.23 55.6,47.48 v55.6,59.82 | K20.6 50.54,11.05 52.07,11.05 | IC6.3 72.39,61.59 72.01,61.21 72.01,58.95 v72.39,58.57 | E7.TP 86.36,70.48 83.44,67.56 v83.44,58.42
  Bottom 0.254: v83.44,58.42 73.81,58.42 R22.2
  Bottom 0.305: v52.07,7.62 R205.2 | v21.59,12.06 v31.75,12.06 v41.91,12.06 v52.07,12.06 | R22.2 v72.39,58.57 R21.1 71.09,58.54 61.6,58.54 60.33,59.82 v55.6,59.82
E8  (via drill 0.35)
  Top 0.254: v72.39,50.16 IC7.6 | v76.49,50.28 76.49,51.47 77.47,52.45 C6.- | 77.47,58.42 v77.47,59.05 | v84.1,59.05 84.1,67.31 84.1,67.59 87.63,71.12 v87.63,76.2
  Top 0.305: C6.- 77.47,58.42
  Bottom 0.254: D1.2 v72.39,50.16 | v72.39,50.16 72.5,50.28 v76.49,50.28 | R14.1 53.34,51.18 53.57,50.95 57.6,50.95 58.08,50.48 69.6,50.48 IC7.6 v72.39,50.16 | v77.47,59.05 v84.1,59.05 | v87.63,76.2 91.44,76.2
  Bottom 0.305: 91.44,76.2 92.71,77.47 E8.TP
E9  (via drill 0.35)
  Top 0.305: IC8.3 116.76,56.53 v115.08,56.53 | v107.82,55.88 R30.3
  Bottom 0.305: E9.TP 107.7,78.74 R30.3 | v115.08,56.53 113.56,56.53 112.9,55.88 v107.82,55.88
E11  (via drill 0.35)
  Top 0.254: v93.98,11.43 v93.98,7.62
  Top 0.305: v86.36,7.62 86.36,10.79 86.06,11.1 K24.3 | E11.TP 119.38,74.93 116.84,72.39 C7.- v116.84,67.31 | v125.73,65.15 126.81,65.15 C8.+ v127,54.61 126.75,54.36 126.75,41.03 129.54,38.23 v129.54,11.43
  Bottom 0.254: 118.2,65.15 116.84,66.51 v116.84,67.31 | v93.98,7.62 v86.36,7.62
  Bottom 0.305: R33.1 v127,54.61 | v125.73,65.15 118.2,65.15 | v129.54,11.43 v93.98,11.43
GND  (via drill 0.35)
  Top 0.254: v55.24,62.72 55.09,62.87 IC2.3 | IC10.13 103.71,38.73 v103.89,38.56 | IC12*.5 57.2,69.22 57.07,69.09 57.07,67.64 v57.27,67.44
  Top 0.305: QS24.2 91.12,18.1 v91.19,18.03 | IC9.13 v103.76,19.68 | IC11.13 6.99,40.01 v6.35,40.64 | IC4.3 89.53,65.41 v90.17,64.77
  Bottom 0.254: C1P.2 39.12,58.29 v38.99,58.42 | C2P.2 55.86,62.1 v55.24,62.72 | C6P.2 v76.97,60.83 v76.96,60.83 | v66.76,51.31 65.99,52.07 C7N.1
  Bottom 0.305: v90.17,64.77 92.58,64.77 C4P.2 | C4N.1 89.41,67.44 v89.54,67.31 | v6.35,40.64 v1.27,40.64 | R10.2 v58.93,48.26 | R35.1 67.16,6.35 v67.31,6.35
  Bottom 0.61: R21.2 v71.12,57.15
  pour Top (isolate 0.406): 0,81.28 167.64,81.28 167.64,0 0,0
  pour Bottom (isolate 0.305): 0,81.28 167.64,81.28 167.64,0 0,0
IC1P5  (via drill 0.35)
  Top 0.305: IC1.5 42.16,57.78 42.42,57.53 v42.42,56.39 | C1.2 44.45,63.5 v44.45,56.39
  Bottom 0.254: v42.42,56.39 v44.45,56.39
IC2P5  (via drill 0.35)
  Top 0.254: v60.2,60.86 60.2,61.21 59.82,61.59 IC2.5
  Bottom 0.254: v60.2,60.86 61.82,60.86 62.23,60.45 C2.2
IC4P5  (via drill 0.35)
  Top 0.305: IC4.5 v94.49,64.14 | v97.79,63.88 C3.2
  Bottom 0.305: v97.79,63.88 97.54,64.14 v94.49,64.14
IC6.6  (via drill 0.35)
  Top 0.254: IC6.6.TP 81.28,58.04 v81.28,59.69 81.28,60.96 80.64,61.59 IC6.6
  Bottom 0.254: R18.1 69.7,59.69 80.16,59.69 v81.28,59.69
  Bottom 0.305: R17.2 v81.28,59.69
MAIN_OUT  (via drill 0.35)
  Top 0.305: K24.6 91.44,11.1 90.47,12.06 v89.66,12.06 | v10.16,6.35 v10.16,13.97 | K21.7 62.01,13.3 62.23,13.08 v62.23,12.06 | K22.3 63.2,11.1 v62.23,12.06 | K23.3 73.36,11.1 v72.39,12.06 | v62.23,6.1 v62.23,12.06
  Bottom 0.305: CON3.2 5.08,13.97 v10.16,13.97 | v62.23,12.06 v72.39,12.06 v89.66,12.06 | v10.16,6.35 24.13,6.35 | CON2.TP 24.13,6.35 | 24.13,6.35 30.6,6.35 31.17,6.92 45.4,6.92 46.23,6.1 v62.23,6.1
N$1
  Bottom 0.305: RKM4.2 50.95,72.39 CKM4.1
N$2
  Bottom 0.305: RLN4.2 74.4,72.39 CLN4.1
N$3  (via drill 0.35)
  Top 0.305: K1.3 13.34,34.29 v16.38,34.29
  Bottom 0.305: v16.38,34.29 RF2.1 16.36,33.02 19.2,33.02 RF1.2
N$4
  Top 0.305: IC1.8 39.37,61.59 38.1,62.87 C1.1
N$5  (via drill 0.35)
  Top 0.305: v24.89,31.75 24.89,33.53 24.46,33.96 K2.3 23.17,33.98 v22.1,35.05
  Bottom 0.305: RF3.1 v24.89,31.75 | RF2.2 18.69,35.05 v22.1,35.05
N$6  (via drill 0.35)
  Top 0.305: K20.4 43.49,5.86 v43.94,5.41 | v69.85,4.95 R4.3
  Bottom 0.305: R4.3 R4.2 | v43.94,5.41 44.12,5.23 56.54,5.23 56.89,5.58 57.41,5.58 57.76,5.23 69.57,5.23 v69.85,4.95
N$7  (via drill 0.35)
  Top 0.305: v142.75,59.69 LED1.A
  Bottom 0.305: RLD.2 143.51,58.93 v142.75,59.69
N$8  (via drill 0.35)
  Top 0.305: v31.75,31.75 31.75,33.02 33.02,34.29 33.33,33.98 K3.3
  Bottom 0.305: RF3.2 v31.75,31.75 RF4.1
N$9  (via drill 0.35)
  Top 0.254: IC1.2 33.91,60.33 33.66,60.07 v33.66,58.42 v33.66,51.43 | v47.74,60.96 47.74,68.06 | IC12*.2 v49.66,71.75 v49.66,71.76
  Top 0.305: v48.26,53.34 47.74,53.86 v47.74,60.96 | 47.74,68.06 47.74,70.61 v47.37,70.98
  Bottom 0.254: v33.66,58.42 33.5,58.27 R5.1 | R7.2 48.26,52.07 47.24,51.05 39.37,51.05 38.99,51.43 v33.66,51.43
  Bottom 0.305: R7.2 v48.26,53.34 | v47.74,60.96 47.59,61.11 R6.1 | v49.66,71.76 48.15,71.76 v47.37,70.98
N$11  (via drill 0.35)
  Top 0.254: IC12*.6 59.82,70.48 60.2,70.1 v60.2,68.58
  Top 0.305: IC2.2 51.05,64.14 v50.8,63.88 50.8,68.07 v50.55,68.33
  Bottom 0.305: R39.2 v50.8,63.88 | v50.55,68.33 59.94,68.33 v60.2,68.58
N$13  (via drill 0.35)
  Top 0.305: v41.91,31.75 41.91,33.02 42.85,33.96 K4.3
  Bottom 0.305: RF4.2 v41.91,31.75 RF5.1
N$14  (via drill 0.35)
  Top 0.254: IC2.8 59.82,65.41 v60.2,65.79
  Bottom 0.254: v60.2,65.79 61.59,65.79 62.23,66.42 C2.1
N$15  (via drill 0.35)
  Top 0.254: IC3.3 38.73,50.16 v38.35,50.55 38.35,57.91 38.1,58.17 38.1,62.23 36.83,63.5 v36.83,68.58 | v57.4,50.29 57.4,51.82 v58.93,53.34 | IC34*.3 74.3,69.22 v73.66,68.58
  Bottom 0.254: v38.35,50.55 57.15,50.55 v57.4,50.29 | v73.66,68.58 71.12,68.58 70.43,69.27 50.6,69.27 49.91,68.58 v36.83,68.58
  Bottom 0.305: R10.1 v58.93,53.34 R11.1
N$16  (via drill 0.35)
  Top 0.254: IC34*.1 74.3,71.75 73.03,70.49 v72.39,70.49 | v49.02,69.85 49.02,50.29 48.9,50.16
  Top 0.305: v49.53,49.53 48.9,50.16 IC3.6
  Bottom 0.305: R7.1 48.41,49.53 v49.53,49.53 50.65,49.53 R8.1 | v72.39,70.49 71.76,70.49 71.38,70.11 49.28,70.11 v49.02,69.85
N$17  (via drill 0.35)
  Top 0.305: Q1.G 53.34,54.61 52.07,53.34 Q1*.3 v52.07,48.01
  Bottom 0.254: Q1G.TP 62.1,56.39 61.59,55.88 Q1.G
  Bottom 0.305: R13.1 R14.2 53.34,49.28 v52.07,48.01
N$18  (via drill 0.35)
  Top 0.254: v42.55,54.36 42.55,51.82 42.16,51.44 IC3.2 | v49.63,69.22 49.43,69.02 49.43,57.25 Q1.D
  Top 0.305: Q1.D v50.8,53.34 51.12,53.02 Q1*.2 | v73.66,69.68 74.46,70.48 IC34*.2
  Bottom 0.254: R9.2 42.65,54.46 v42.55,54.36 | v73.66,69.68 50.09,69.68 v49.63,69.22
  Bottom 0.305: R8.2 v50.8,53.34 50.16,53.98 48.11,53.98 47.63,54.46 R9.2 | Q1.D 51.82,55.88 53.24,57.3 R12.1
N$20  (via drill 0.35)
  Top 0.254: IC34*.6 82.8,69.22 83.19,68.83 83.19,67.92 83.01,67.74 83.01,67.41 v82.79,67.19
  Top 0.305: IC4.2 85.72,66.67 v85.09,67.31
  Bottom 0.305: v85.09,67.31 84.96,67.44 R40.2 83.04,67.44 v82.79,67.19
N$21
  Top 0.305: QS11.1 129.4,43.18 RS11.1
N$23  (via drill 0.35)
  Top 0.254: v78.74,54.61 78.74,49.53 77.66,49.53 C6.+
  Bottom 0.254: v78.74,54.61 78.36,54.23 R15.1
N$24  (via drill 0.35)
  Top 0.254: v81.28,49.53 81.28,54.74 82.68,56.13 v82.68,63.63
  Bottom 0.254: D3.2 D2.1 80.44,49.53 v81.28,49.53 82.4,49.53 R16.2 | v82.68,63.63 81.31,63.63 R17.1
N$25  (via drill 0.35)
  Top 0.254: IC7.2 63.37,51.44 62.87,51.94 62.87,54.36 v63.12,54.61
  Bottom 0.254: v63.12,54.61 63.5,54.23 R15.2 65.15,54.23 66.33,53.05 71.84,53.05 D1.1
  Bottom 0.305: R16.1 82.27,52.5 D2.2 D3.1 D1.1
N$27  (via drill 0.35)
  Top 0.305: v69.85,63.5 70.48,62.87 IC6.2
  Bottom 0.305: R19.1 70,63.65 v69.85,63.5 69.7,63.65 R18.2 R20.1
N$28  (via drill 0.35)
  Top 0.305: v52.07,31.75 52.07,32.89 53.14,33.96 K5.3
  Bottom 0.305: RF5.2 v52.07,31.75 RF6.1
N$30
  Top 0.305: Q4.3 101.6,57.15 100.33,58.42 100.33,60.96 101.6,62.23 Q3.3
  Bottom 0.305: R22.1 82.7,55.73 85.09,53.34 90.17,53.34 91.44,54.61 Q4.3
N$31  (via drill 0.35)
  Top 0.254: C5.+ R27.1
  Bottom 0.305: R27.1 102.39,56.03 Q4.2
  other vias: 96.52,56.03
N$32
  Top 0.305: RS24.1 87.59,19.22 QS24.1
N$33  (via drill 0.35)
  Top 0.305: v92.84,51.56 94.74,51.56 | 94.74,51.56 96.17,51.56 C5.- | IC5.6 94.11,47.62 94.74,48.26 94.74,51.56
  Bottom 0.305: R25.1 92.84,53.06 v92.84,51.56
N$34  (via drill 0.35)
  Top 0.254: v95.25,53.34 v95.25,58.42
  Top 0.305: Q2.1 102.87,60.96 Q2.2
  Bottom 0.254: R27.2 96.37,53.34 v95.25,53.34 | v95.25,58.42 95.4,58.27 R26.1 R28.1 102.72,58.27 Q2.1
N$35  (via drill 0.35)
  Top 0.305: v76.2,10.16 76.2,9.4 75.69,8.89 75.68,8.9 K23.4
  Bottom 0.305: R36.2 R35.2 76.05,10.31 v76.2,10.16 R34.2
N$36  (via drill 0.35)
  Top 0.305: v65.41,31.75 65.41,33.53 64.97,33.96 K6.3
  Bottom 0.305: RF6.2 v65.41,31.75 RF7.1
N$37  (via drill 0.35)
  Top 0.305: v72.39,31.75 72.39,33.02 73.33,33.96 K7.3
  Bottom 0.305: RF7.2 v72.39,31.75 RF8.1
N$38  (via drill 0.35)
  Top 0.305: v82.55,31.75 82.55,33.15 83.36,33.96 K8.3
  Bottom 0.305: RF8.2 v82.55,31.75 RF9.1
N$39  (via drill 0.35)
  Top 0.305: K9.3 106.76,33.96 107.31,33.4 v107.31,31.62
  Bottom 0.305: RF9.2 90.45,31.62 v107.31,31.62 108.94,31.62 RF10.1
N$40  (via drill 0.35)
  Top 0.305: v114.3,31.75 114.3,32.89 115.37,33.96 K10.3
  Bottom 0.305: RF10.2 v114.3,31.75 RF11.1
N$41  (via drill 0.35)
  Top 0.305: K1.6 20.34,34.29 v21.59,34.29 v21.59,29.21
  Bottom 0.305: v21.59,34.29 RE2.1 | RE1.2 17.17,29.21 v21.59,29.21
N$42  (via drill 0.35)
  Top 0.305: K2.6 31.42,33.96 v31.75,34.29
  Bottom 0.305: RE3.1 v31.75,34.29 RE2.2
N$43  (via drill 0.35)
  Top 0.305: K3.6 41.58,33.96 v41.91,34.29
  Bottom 0.305: RE4.1 v41.91,34.29 RE3.2
N$44  (via drill 0.35)
  Top 0.305: v52.07,34.29 51.74,33.96 K4.6
  Bottom 0.305: RE4.2 v52.07,34.29 RE5.1
N$45  (via drill 0.35)
  Top 0.305: v60.71,34.92 60.71,34.02 K5.6
  Bottom 0.305: RE5.2 57.94,34.92 v60.71,34.92 63.98,34.92 RE6.1
N$46  (via drill 0.35)
  Top 0.305: v72.39,34.29 71.14,34.29 K6.6
  Bottom 0.305: RE6.2 v72.39,34.29 RE7.1
N$47  (via drill 0.35)
  Top 0.305: v82.55,34.29 81.3,34.29 K7.6
  Bottom 0.305: RE7.2 v82.55,34.29 RE8.1
N$48  (via drill 0.35)
  Top 0.305: v92.71,34.29 91.46,34.29 K8.6
  Bottom 0.254: v92.71,34.29 93.98,33.02 104.14,33.02 105.41,34.29 RE9.1
  Bottom 0.305: RE8.2 v92.71,34.29
N$49  (via drill 0.35)
  Top 0.305: v114.3,34.29 113.05,34.29 K9.6
  Bottom 0.305: RE9.2 v114.3,34.29 RE10.1
N$50  (via drill 0.35)
  Top 0.305: v122.81,35.05 122.81,34.03 K10.6
  Bottom 0.305: RE10.2 120.29,35.05 v122.81,35.05 126.09,35.05 RE11.1
N$51
  Top 0.305: QS1.1 17,43.18 RS1.1
N$52  (via drill 0.35)
  Top 0.508: v18.54,39.37 18.55,39.36 19.05,39.36 | 19.05,39.36 K1.8 | QS1.3 19.05,39.36
  Bottom 0.508: DS1.A 18.56,39.35 v18.54,39.37
N$53
  Top 0.305: QS2.1 27.16,43.18 RS2.1
N$54  (via drill 0.35)
  Top 0.508: v28.7,39.37 28.71,39.36 29.21,39.36 | 29.21,39.36 K2.8 | QS2.3 29.21,39.36
  Bottom 0.508: DS2.A 28.72,39.35 v28.7,39.37
N$55
  Top 0.305: QS3.1 37.32,43.18 RS3.1
N$56  (via drill 0.35)
  Top 0.508: v38.86,39.37 38.87,39.36 39.37,39.36 | 39.37,39.36 K3.8 | QS3.3 39.37,39.36
  Bottom 0.508: DS3.A 38.88,39.35 v38.86,39.37
N$57
  Top 0.305: QS4.1 47.48,43.18 RS4.1
N$58  (via drill 0.35)
  Top 0.508: v49.02,39.37 49.03,39.36 49.53,39.36 | 49.53,39.36 K4.8 | QS4.3 49.53,39.36
  Bottom 0.508: DS4.A 49.04,39.35 v49.02,39.37
N$59
  Top 0.305: QS5.1 57.13,43.18 RS5.1
N$60  (via drill 0.35)
  Top 0.508: v59.18,39.37 59.19,39.36 | 59.19,39.36 59.69,39.36 K5.8 | 59.19,39.36 v59.18,39.36 QS5.3
  Bottom 0.508: DS5.A 59.2,39.35 v59.18,39.37
N$61
  Top 0.305: QS6.1 67.8,43.18 RS6.1
N$62  (via drill 0.35)
  Top 0.508: v69.34,39.37 69.85,39.37 | 69.85,39.37 K6.8 | QS6.3 69.85,39.37
  Bottom 0.508: DS6.A 69.34,36.85 v69.34,39.37
N$63
  Top 0.305: QS7.1 77.58,43.18 RS7.1
N$64  (via drill 0.35)
  Top 0.508: v79.5,39.37 80.01,39.37 | 80.01,39.37 K7.8 | QS7.3 80.01,39.37
  Bottom 0.508: DS7.A 79.52,39.35 v79.5,39.37
N$65
  Top 0.305: QS8.1 87.87,43.18 RS8.1
N$66  (via drill 0.35)
  Top 0.508: v89.66,39.37 90.17,39.37 | 90.17,39.37 K8.8 | QS8.3 90.17,39.37
  Bottom 0.508: DS8.A 89.68,39.35 v89.66,39.37
N$67
  Top 0.305: QS9.1 109.71,43.18 RS9.1
N$68  (via drill 0.35)
  Top 0.508: v111.25,39.37 111.76,39.37 | 111.76,39.37 K9.8 | QS9.3 111.76,39.37
  Top 0.61: K9.8
  Bottom 0.508: DS9.A 111.27,39.35 v111.25,39.37
N$69
  Top 0.305: QS10.1 119.87,43.18 RS10.1
N$70  (via drill 0.35)
  Top 0.508: v121.41,39.24 121.92,39.24 | 121.92,39.24 122.76,39.24 K10.8 | QS10.3 121.92,39.24
  Bottom 0.508: DS10.A 121.43,39.23 v121.41,39.24
N$71
  Top 0.305: IC4.8 95.25,67.94 95.89,67.94 97.28,67.94 97.79,68.45 C3.1
N$72  (via drill 0.35)
  Top 0.305: K11.3 126.95,33.96 127.25,33.66 127.25,26.92 v127,26.67
  Bottom 0.305: CKM1.1 123.19,26.67 v127,26.67
N$73  (via drill 0.35)
  Top 0.305: K12.3 136.85,33.96 137.48,33.34 137.67,33.15 v137.67,24.13
  Bottom 0.305: v137.67,24.13 CKM2.1
N$74
  Top 0.305: K13.3 147.14,33.96 147.83,33.27 147.83,28.45 CKM3.2
N$75  (via drill 0.35)
  Top 0.508: K11.8 v131.57,39.37 131.44,39.5 QS11.3
  Bottom 0.508: DS11.A 131.59,39.35 v131.57,39.37
N$76  (via drill 0.35)
  Top 0.305: v95.25,62.21 95.43,62.38 C4.+ 97.31,62.38 101.6,66.67 Q3.2
  Bottom 0.305: v95.25,62.21 96.34,61.11 R26.2
N$77
  Top 0.305: QS12.1 140.19,43.18 RS12.1
N$78  (via drill 0.35)
  Top 0.508: v141.73,39.37 142.24,39.37 | 142.24,39.37 K12.8 | QS12.3 142.24,39.37
  Bottom 0.508: DS12.A 141.75,39.35 v141.73,39.37
N$79
  Top 0.305: QS13.1 150.35,43.18 RS13.1
N$80  (via drill 0.35)
  Top 0.508: v151.89,39.37 152.4,39.37 | 152.4,39.37 K13.8 | QS13.3 152.4,39.37
  Bottom 0.508: DS13.A 151.91,39.35 v151.89,39.37
N$81
  Top 0.305: QS14.1 160.51,43.18 RS14.1
N$82  (via drill 0.35)
  Top 0.508: v162.05,39.37 162.56,39.37 | 162.56,39.37 K14.8 | QS14.3 162.56,39.37
  Bottom 0.508: DS14.A 162.07,39.35 v162.05,39.37
N$83  (via drill 0.35)
  Top 0.305: K17.5 v21.58,8.9 v21.59,8.89 | v25.21,8.19 26.29,7.1 v26.29,4.06
  Bottom 0.254: 38.1,3.4 38.15,3.45 99.28,3.45 100.5,4.67 101.77,4.67 102.17,5.08 C9.1
  Bottom 0.305: v21.59,8.89 R43.2 24.51,8.89 v25.21,8.19 | 38.1,3.4 36.74,3.4 36.28,3.86 26.5,3.86 v26.29,4.06
N$84  (via drill 0.35)
  Top 0.305: K19.4 34.29,7.94 v34.29,5.2 | v57.15,4.95 R3.3
  Bottom 0.305: R3.3 R3.2 | v34.29,5.2 41.79,5.2 42.22,4.78 56.98,4.78 v57.15,4.95
N$85  (via drill 0.35)
  Top 0.305: K17.4 v15.23,8.9 v15.24,8.89 | v30.48,7.49 R1.3
  Bottom 0.305: v15.24,8.89 16.64,7.49 v30.48,7.49 | R1.3 R1.2
N$86  (via drill 0.35)
  Top 0.305: v25.65,3.56 25.65,5.84 24.51,6.99 24.51,8.51 24.12,8.9 K18.4
  Bottom 0.305: R2.2 R2.3 38.1,2.54 37.85,2.54 36.96,2.54 36.09,3.4 25.81,3.4 v25.65,3.56
N$87  (via drill 0.35)
  Top 0.254: C10.1 v114.3,7.62
  Top 0.305: K18.5 v31.74,8.9 v31.75,8.89 v31.75,4.57
  Bottom 0.254: 36.93,3.86 99.11,3.86 100.33,5.08 101.6,5.08 102.87,6.35 106.68,6.35 107.95,7.62 v114.3,7.62
  Bottom 0.305: R43.1 v31.75,8.89 R42.2 | v31.75,4.57 36.22,4.57 36.93,3.86
N$88  (via drill 0.35)
  Top 0.254: C11.1 100.33,5.08 v100.33,6.32
  Top 0.305: v38.73,8.89 K19.5 v40.33,4.52 v40.33,4.51
  Bottom 0.254: 72.39,4.32 98.33,4.32 v100.33,6.32
  Bottom 0.305: R42.1 v38.73,8.89 R41.2 | 72.39,4.32 40.52,4.32 v40.33,4.51
N$89  (via drill 0.35)
  Top 0.254: v107.95,8.89 C12.1
  Top 0.305: v48.9,8.89 v48.91,8.9 K20.5
  Bottom 0.254: v107.95,8.89 106.07,7.01 69.19,7.01 67.31,8.89
  Bottom 0.305: R41.1 v48.9,8.89 67.31,8.89
N$90
  Top 0.305: RS18.1 26.63,19.22 QS18.1
N$91  (via drill 0.35)
  Top 0.508: v28.7,16.51 28.71,16.5 29.21,16.5 | 29.21,16.5 K18.8 | QS18.3 29.21,16.5
  Bottom 0.508: DS18.A 28.72,16.49 v28.7,16.51
N$92
  Top 0.305: RS19.1 36.79,19.22 QS19.1
N$93  (via drill 0.35)
  Top 0.508: v38.86,16.51 38.87,16.5 39.37,16.5 | 39.37,16.5 K19.8 | QS19.3 39.37,16.5
  Bottom 0.508: DS19.A 38.88,16.49 v38.86,16.51
N$94
  Top 0.305: RS20.1 46.95,19.22 QS20.1
N$95  (via drill 0.35)
  Top 0.508: v49.02,16.51 49.53,16.51 | 49.53,16.51 K20.8 | QS20.3 49.53,16.51
  Bottom 0.508: DS20.A 49.04,16.49 v49.02,16.51
N$96  (via drill 0.35)
  Top 0.305: K21.3 54.94,11.1 55.24,10.79 v55.24,7.62
  Bottom 0.305: v55.24,7.62 R205.1
N$97
  Bottom 0.305: R23.1 92.56,58.42 90.17,58.42 88.9,59.69 R24.1
N$98  (via drill 0.35)
  Top 0.305: v63.5,7.62 63.81,7.93 K22.4
  Bottom 0.305: R37.2 R36.1 61.11,7.62 v63.5,7.62
N$99  (via drill 0.35)
  Top 0.305: K24.4 v85.72,8.9 v85.72,8.89
  Bottom 0.305: v85.72,8.89 85.83,8.99 R38.1
N$100  (via drill 0.35)
  Top 0.305: K24.5 v88.9,8.89
  Bottom 0.305: v88.9,8.89 88.67,9.12 R38.2
N$101  (via drill 0.35)
  Top 0.305: v82.55,10.16 82.55,12.7 83.15,13.3 K24.2
  Bottom 0.305: R34.1 v82.55,10.16
N$102  (via drill 0.35)
  Top 0.254: v110.49,49.53 110.49,75.95 R30.2
  Top 0.305: K14.3 155.4,33.96 154.94,34.42 v154.94,49.53
  Bottom 0.254: v154.94,49.53 v110.49,49.53
  Bottom 0.305: R29.1 108.08,73.79 R30.2
N$103
  Top 0.305: RS21.1 57.11,19.22 QS21.1
N$104  (via drill 0.35)
  Top 0.508: v59.18,16.51 59.19,16.5 59.69,16.5 | 59.69,16.5 K21.8 | QS21.3 59.69,16.5
  Bottom 0.508: DS21.A 59.2,16.49 v59.18,16.51
N$105
  Top 0.305: RS22.1 67.27,19.22 QS22.1
N$106  (via drill 0.35)
  Top 0.508: v69.34,16.51 69.35,16.5 69.85,16.5 | 69.85,16.5 K22.8 | QS22.3 69.85,16.5
  Bottom 0.508: DS22.A 69.36,16.49 v69.34,16.51
N$107
  Top 0.305: RS23.1 77.43,19.22 QS23.1
N$108  (via drill 0.35)
  Top 0.508: v79.5,16.51 80.01,16.51 | 80.01,16.51 K23.8 | QS23.3 80.01,16.51
  Bottom 0.508: DS23.A 79.5,13.99 v79.5,16.51
N$109  (via drill 0.35)
  Top 0.508: v89.66,16.51 90.17,16.51 | 90.17,16.51 K24.8 | QS24.3 90.17,16.51
  Bottom 0.508: DS24.A 89.68,16.49 v89.66,16.51
N$110
  Top 0.305: RS17.1 14.94,19.22 QS17.1
N$111  (via drill 0.35)
  Top 0.508: v18.54,16.51 18.55,16.5 19.05,16.5 | 19.05,16.5 K17.8 | QS17.3 19.05,16.5
  Bottom 0.508: DS17.A 18.56,16.49 v18.54,16.51
N$112  (via drill 0.35)
  Top 0.305: IC9.9 101.5,15.24 100.48,15.24 99.04,16.69 v99.04,39.37 | v103.89,39.37 103.89,39.75 103.63,40.01 IC10.14
  Bottom 0.305: v99.04,39.37 v103.89,39.37
N$113  (via drill 0.35)
  Top 0.305: IC10.9 v100.61,33.66 | IC11.14 v7.75,41.27 | v99.04,42.34 98.41,41.7 v98.41,33.66
  Bottom 0.305: v98.41,33.66 v100.61,33.66 | v7.75,41.27 8.89,41.27 11.35,43.74 62.43,43.74 63.6,42.57 98.8,42.57 v99.04,42.34
N$114  (via drill 0.35)
  Top 0.305: K11.6 131.88,33.96 131.57,33.66 v131.57,25.4
  Bottom 0.305: v131.57,25.4 CLN1.1
N$115
  Top 0.305: CLN2.1 139.19,31.37 141.73,33.91 143.15,33.91 K12.6
N$116
  Top 0.305: CLN3.2 151.13,32.89 152.2,33.96 K13.6
N$117
  Bottom 0.305: R24.3 89.05,56.03 R25.2
N$118
  Top 0.305: IC5.2 86.23,48.9 85.72,49.4 85.72,56.52 86.36,57.15 R24.2
N$120  (via drill 0.35)
  Top 0.254: C7.+ 118.78,64.96 v120.37,66.55 | IC8.6 123.83,56.52 124.46,57.15 v124.46,66.55 124.46,68.58 125.73,69.85 127,69.85 C8.-
  Bottom 0.254: v120.37,66.55 120.4,66.57 R32.2 124.44,66.57 v124.46,66.55
N$121  (via drill 0.35)
  Top 0.254: 119.51,57.15 119.51,63.63 v119.63,63.75
  Top 0.305: v115.08,57.78 IC8.2 119,57.78 119.51,57.28 119.51,57.15 v119.51,54.61
  Bottom 0.254: v119.63,63.75 119.66,63.73 R32.1
  Bottom 0.305: v115.08,57.78 114.6,57.3 R31.2
R01  (via drill 0.35)
  Top 0.305: IC11.7 v1.78,36.2 | v12.57,41.1 RS1.2
  Bottom 0.305: v1.78,36.2 7.04,36.2 11.95,41.1 v12.57,41.1
R02  (via drill 0.35)
  Top 0.305: IC11.6 v1.78,37.47 | v22.73,41.73 RS2.2
  Bottom 0.305: v1.78,37.47 7.67,37.47 11.94,41.73 12.62,41.73 12.7,41.73 v22.73,41.73
R03  (via drill 0.35)
  Top 0.305: IC11.5 v1.78,38.73 | v31.37,42.19 32.36,43.18 RS3.2
  Bottom 0.305: v1.78,38.73 8.29,38.73 8.91,39.35 11.92,42.37 31.19,42.37 v31.37,42.19
R04  (via drill 0.35)
  Top 0.305: IC11.4 v1.78,40.01 | v41.4,42.65 41.93,43.18 RS4.2
  Bottom 0.305: v1.78,40.01 8.91,40.01 11.73,42.82 41.23,42.82 v41.4,42.65
R05  (via drill 0.35)
  Top 0.305: IC11.3 v1.78,41.27 | v51.69,43.11 51.76,43.18 RS5.2
  Bottom 0.305: v1.78,41.27 6.85,41.27 7.49,40.64 8.9,40.64 11.54,43.28 51.51,43.28 v51.69,43.11
R06  (via drill 0.35)
  Top 0.305: IC11.2 v1.78,42.55 | RS6.2 64.13,43.94 v64.52,43.94
  Bottom 0.305: v1.78,42.55 6.85,42.55 7.49,41.91 8.77,41.91 11.05,44.2 64.26,44.2 v64.52,43.94
R07  (via drill 0.35)
  Top 0.305: RS7.2 73.53,43.43 v72.14,44.83 | v1.78,43.81 IC11.1
  Bottom 0.305: v1.78,43.81 3.3,43.81 3.87,43.24 6.41,43.24 6.47,43.18 8.64,43.18 10.57,45.11 70.97,45.11 71.25,44.83 v72.14,44.83
R08  (via drill 0.35)
  Top 0.305: IC11.15 v7.75,42.55 | RS8.2 82.67,44.2 v82.3,44.2
  Bottom 0.305: v7.75,42.55 7.93,42.73 8.83,42.73 10.76,44.65 70.78,44.65 71.23,44.2 v82.3,44.2
R09  (via drill 0.35)
  Top 0.254: IC10.7 92.58,34.92 92.33,35.18 v92.33,44.45 | v106.05,44.45 RS9.2
  Bottom 0.254: v92.33,44.45 100.27,44.45 100.96,45.15 103.13,45.15 103.82,44.45 v106.05,44.45
R10  (via drill 0.35)
  Top 0.254: IC10.6 93.09,36.2 92.73,36.55 92.73,43.46 93.22,43.94 v93.22,45.06 | v115.32,44.83 115.44,44.71 RS10.2
  Bottom 0.254: v93.22,45.06 93.42,44.86 100.1,44.86 100.79,45.55 103.3,45.55 103.95,44.9 105.63,44.9 105.79,45.06 115.09,45.06 v115.32,44.83
R11  (via drill 0.35)
  Top 0.254: RS17.2 v13.97,26.85 | v97.79,26.85 97.79,36.96 97.28,37.47 IC10.5
  Bottom 0.254: v13.97,26.85 14.17,27.05 97.59,27.05 v97.79,26.85
R12  (via drill 0.35)
  Top 0.254: IC10.4 94.11,38.73 93.64,39.2 v93.64,41.91 | RS18.2 v22.73,26.44 | v109.22,26.67 109.22,40.32 v107.79,41.75
  Bottom 0.254: v22.73,26.44 22.93,26.64 97.14,26.64 97.54,26.24 98.04,26.24 98.47,26.67 v109.22,26.67 | v107.79,41.75 107.77,41.73 98.2,41.73 97.79,42.14 94.11,42.14 93.88,41.91 v93.64,41.91
R13  (via drill 0.35)
  Top 0.254: v97.77,41.09 97.77,40.12 97.66,40.01 IC10.3 | v34.37,40.98 35.41,39.95 35.41,30.83 33.02,28.45 33.02,20.45 RS19.2
  Bottom 0.254: v34.37,40.98 34.51,40.84 93.98,40.84 94.33,40.84 97.52,40.84 v97.77,41.09
R14  (via drill 0.35)
  Top 0.254: v46.22,41.45 46.22,25.14 43.18,22.1 43.18,20.45 RS20.2 | IC10.2 94.61,41.27 v94.36,41.53
  Bottom 0.254: v94.36,41.53 94.12,41.53 93.9,41.3 46.37,41.3 v46.22,41.45
R15  (via drill 0.35)
  Top 0.254: IC10.1 97.54,42.55 97.92,42.93 v97.92,48.26 v97.91,48.26
  Top 0.305: RS11.2 125.73,43.31 v125.73,48.26
  Bottom 0.305: v125.73,48.26 v97.91,48.26
R16  (via drill 0.35)
  Top 0.305: IC10.15 103.8,41.27 v104.14,40.94 | v135.76,41.02 RS12.2
  Bottom 0.305: v104.14,40.94 104.22,41.02 v135.76,41.02
R17  (via drill 0.35)
  Top 0.305: RS13.2 148.59,40.51 v148.59,15.24 | v93.85,15.88 IC9.7
  Bottom 0.305: v148.59,15.24 118.11,15.24 116.84,16.51 94.49,16.51 v93.85,15.88
R20  (via drill 0.35)
  Top 0.305: IC9.4 v93.98,19.68 | RS14.2 156.08,42.8 158.75,40.13 v158.75,21.46
  Bottom 0.305: v93.98,19.68 98.3,19.68 98.93,20.32 105.66,20.32 106.81,21.46 v158.75,21.46
R21  (via drill 0.35)
  Top 0.305: v53.21,23.62 RS21.2 | IC9.3 93.64,20.95 92.81,21.79 v92.81,24.08
  Bottom 0.305: v53.21,23.62 53.42,23.82 92.55,23.82 v92.81,24.08
R22  (via drill 0.35)
  Top 0.305: RS22.2 v63.37,23.19 | IC9.2 93.98,22.23 93.73,22.48 v93.73,24.13
  Bottom 0.305: v63.37,23.19 63.55,23.37 93.58,23.37 93.73,23.51 v93.73,24.13
R23  (via drill 0.35)
  Top 0.305: IC9.1 v94.36,23.5 | v73.53,22.74 v73.53,22.73 RS23.2
  Bottom 0.305: v73.53,22.74 73.71,22.91 88.9,22.91 89.1,22.91 93.77,22.91 v94.36,23.5
R24  (via drill 0.35)
  Top 0.305: IC9.15 v103.76,22.23 | v83.69,22.23 v83.69,22.22 RS24.2
  Bottom 0.305: v103.76,22.23 v83.69,22.23
SDIN  (via drill 0.35)
  Top 0.305: IC9.14 v103.76,20.95
  Bottom 0.305: v103.76,20.95 8.26,20.95 7.62,21.59 5.08,21.59 CON3.8
SHCP  (via drill 0.35)
  Top 0.305: IC10.11 103.63,36.2 103.94,35.89 103.94,28.57 | IC9.11 103.63,17.14 104.39,17.9 104.39,22.48 104.39,22.49 104.02,22.86 103.94,22.94 103.94,28.57 | IC11.11 7.62,37.47 6.99,36.83 v6.99,27.94 | CON3.7 6.99,23.5 v6.99,27.94 | v103.25,28.58 v103.25,28.57 103.94,28.57 | v6.99,27.94 v6.98,27.94
  Bottom 0.305: v6.98,27.94 102.61,27.94 v103.25,28.58
STCP  (via drill 0.35)
  Top 0.305: IC10.12 103.63,37.47 104.39,36.7 104.39,27.94 | v105.79,19.18 104.85,20.11 104.85,22.67 104.39,23.13 104.39,27.94 | v103.38,18.41 IC9.12 | CON3.5 5.08,21.59 5.08,24.13 6.35,25.4 v6.35,27.43 6.35,27.68 6.35,37.85 7.24,38.73 IC11.12 | v105.03,27.94 104.39,27.94
  Bottom 0.305: v103.38,18.41 105.03,18.41 v105.79,19.18 | v6.35,27.43 6.6,27.43 6.72,27.31 8,27.31 8.18,27.48 104.57,27.48 v105.03,27.94

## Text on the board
tDocu: POWER / SUPPLY | R(F) | C(KM) | R(E) | C(LN) | LEVEL / POTMETER | MICA | MICA | or LM4562 | or LM4562 | E B C | MICA | MICA | SIGNAL / GENERATOR | THD Analyzer B. Cordell / PCB 1 SIGNAL GENERATOR / PCB by Emile / v0.30, 2024-06 | MICA | S | +15V | GND | -15V | D | G | G | E B C | S | D | MPET | MPET | MPET | MPET | MPET | MICA | MICA | MPET | MPET | MPET | 200 Hz | 2 kHz | 20 kHz | 200 kHz | RELAYS + / DIGITAL LOGIC | SYNC | GND | MAIN OUT
bDocu: THD Analyzer B. Cordell / PCB 1, SIGNAL GENERATOR / PCB by Emile, V0.30 / Bottom-Layer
